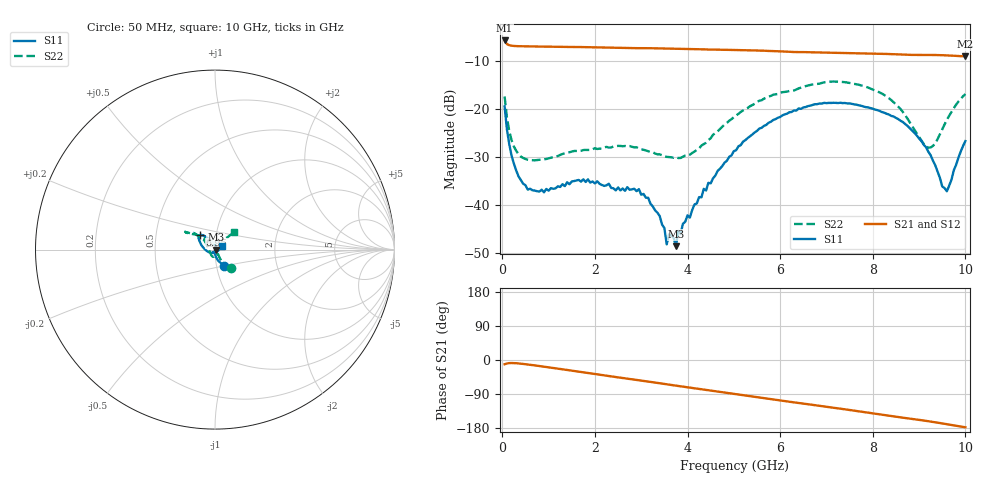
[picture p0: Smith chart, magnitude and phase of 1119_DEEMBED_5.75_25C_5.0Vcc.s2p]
!Hittite Microwave Corp.
!Digital Attenuator/PhaseShifter Rev 1.4.0
!Filename: C:\DATA\DATA\1119_DEEMBED_5.75_25C_5.0Vcc.s2p
!VNA ID: Agilent Technologies,N5224A,MY51441122,A.10.45.03
!Device type:
!2 Port Calibration.
!Temp(C): 25
!Lot Number:
!Serial Number:
!Operator:
!Misc:
!Attenuator:  5.750
# GHZ S DB R 50.0
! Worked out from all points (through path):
!   200 points, 50 MHz to 10 GHz, reference 50 ohm
!   highest |S21| = -5.67 dB at 50 MHz (marker M1); lowest = -9.0 dB at 10 GHz (marker M2)
!   group delay of S21, straight-line fit = 48 ps
!   lowest |S11| = -48.7 dB at 3.75 GHz (marker M3), VSWR 1.01, Z = 50.4 - j0.0247 ohm
!   |S11| at or under -10 dB: start of sweep to end of sweep
!   |S22| runs from -30.7 to -14.2 dB; largest |S21 - S12| = 0.0011
!   S11 on the Smith chart (normalised r, x): 50 MHz: 1.09, -0.21; 6.95 GHz: 0.84, +0.14; 10 GHz: 1.08, +0.05
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0.05  -19.44 -61.3  -5.67 -11.2  -5.66 -11.2  -17.38 -49.1
0.1  -24.25 -75.3  -6.43 -9.3  -6.43 -9.3  -21.74 -59.0
0.2  -29.73 -86.4  -6.76 -8.0  -6.77 -8.0  -26.51 -60.3
0.55  -36.84 -102.1  -6.91 -11.8  -6.91 -11.8  -30.59 -55.4
1.75  -34.68 -118.5  -7.06 -32.5  -7.06 -32.5  -28.57 -80.4
2.95  -36.74 -99.6  -7.27 -53.4  -7.28 -53.4  -28.27 -119.3
3.4  -42.38 -88.4  -7.32 -61.4  -7.33 -61.4  -29.49 -136.9
3.5  -44.88 -74.6  -7.33 -63.2  -7.34 -63.2  -29.91 -141.8
3.55  -48.28 -57.6  -7.34 -64.2  -7.35 -64.2  -30.00 -143.2
3.6  -46.16 -42.8  -7.37 -65.1  -7.38 -65.1  -30.04 -146.0
3.75  -48.66 -3.8  -7.39 -67.7  -7.40 -67.7  -30.09 -155.4
3.8  -45.47 -4.4  -7.40 -68.6  -7.40 -68.6  -30.24 -159.4
3.85  -46.14 13.4  -7.42 -69.4  -7.42 -69.5  -30.23 -162.6
4.35  -36.68 61.2  -7.54 -78.0  -7.55 -78.1  -27.35 159.0
5.05  -28.60 101.1  -7.66 -90.2  -7.68 -90.2  -21.33 138.4
5.85  -22.29 123.7  -7.89 -104.4  -7.90 -104.5  -17.01 141.3
6.7  -19.16 132.8  -8.15 -118.4  -8.16 -118.4  -14.87 147.9
6.95  -18.71 135.2  -8.21 -122.4  -8.22 -122.5  -14.42 149.5
8.35  -21.15 156.7  -8.51 -146.9  -8.51 -146.9  -17.75 140.8
9.2  -28.93 -155.3  -8.70 -161.5  -8.71 -161.6  -28.07 106.7
9.6  -37.18 -59.0  -8.79 -169.4  -8.80 -169.4  -22.26 49.5
10  -26.70 29.6  -9.01 -177.6  -9.02 -177.6  -16.88 42.5
